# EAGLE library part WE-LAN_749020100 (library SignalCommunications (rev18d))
LAN-Transformer WE-LAN 10/10/1000 Base Tx - Compliant with IEEE 802.3 standards - SMD -- Ethernet -- Power over Ethernet -- 1 Gigabit Ethernet -- Compliant with most IC's for ethernet applications like Intel, AMD, Globespan and Realtek -- Hub, Router, Switch Details see: http://katalog.we-online.de/en/pbs/WE-LAN/S/749020100? Updated by Dan Xu 2014-07-08 2014 (C) Würth Elektronik
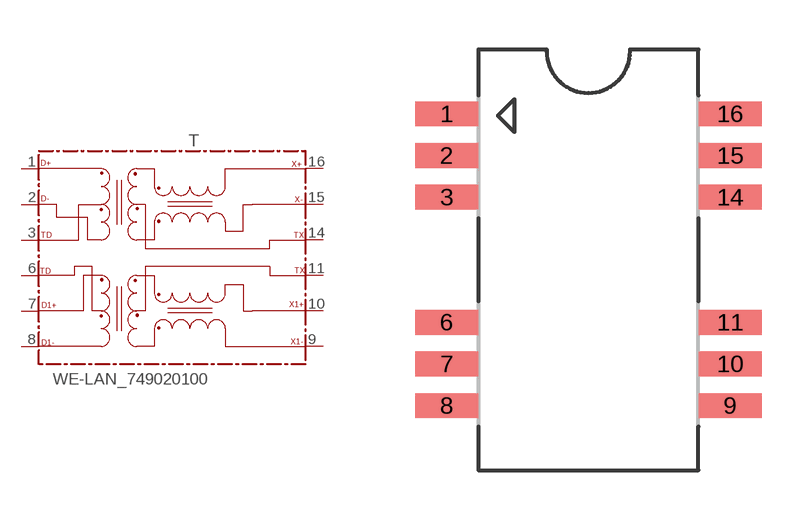
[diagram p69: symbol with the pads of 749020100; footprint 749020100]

Designator prefix T

## WE-LAN_749020100  [749020100]
1  D+
2  D-
3  TD1
6  TD2
7  D1+
8  D1-
9  X1-
10  X1+
11  TX1
14  TX
15  X-
16  X+

## Footprint 749020100 (pad centres in mm)
MAX Height = 2.16mm
smd 1.91 x 0.76: 1 -4.315,4.445; 2 -4.315,3.175; 3 -4.315,1.905; 6 -4.315,-1.905; 7 -4.315,-3.175; 8 -4.315,-4.445; 9 4.315,-4.445; 10 4.315,-3.175; 11 4.315,-1.905; 14 4.315,1.905; 15 4.315,3.175; 16 4.315,4.445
